| TEXAS INSTRUMENTS INCORPORATED
| Standard Linear and Logic Group
| IBIS Model of SN74AUC16244
| 16-Bit Bufer/Driver with 3-State Outputs
| This file contains package information for the following:
|  TSSOP 48-pin (DGG) package as [Component] AUC16244_DGG
|  TVSOP 48-pin (DGV) package as [component] AUC16244_DGV
|  VFBGA 56-PIN (GQL) PACKAGE AS [COMPONENT] AUC16244-GQL
| This device can be powered at the following Vccs:
|  2.5 volt Vcc
|  1.8 volt Vcc
|  1.5 volt Vcc
|  1.2 volt Vcc
|  0.8 volt Vcc
| This file provides unique models under the [Model Selector] for each Vcc.
| For operation at a specific Vcc, select the appropriate model after each
| [Model Selector] keyword.
[IBIS Ver]   3.2
[Comment char]  |_char
[File Name]   sn74auc16244.ibs
[File Rev]   1.1 | x_die
[Date]   May 23, 2002
[Source]   Data created from TI-SPICE simulations at TI-SLL.
[Notes]   The following is an IBIS list for the AUC16244.
   Please contact sllibis@ti.com with questions and
   comments concerning SLL IBIS models.
   -Power clamp data deleted as there is no power-clamp diode.
   -The waveforms for the AUC16244_OUT ,Pullup and
   Pulldown are caused by the circuitry that helps reduce
   overshoot and undershoot in transmission lines (EMI).
   These waveforms are norimal for this particular design.
   -End point warning due to AC and DC mismatch.
   -GQL package is package preview only at this date
[Disclaimer] Property of Texas Instruments Incorporated.  Unauthorized
   reproduction and/or distribution is strictly prohibited.
   This product is protected under copyright law.
   Created  2002, (C) Copyright  2002, Texas Instruments
   Incorporated, All Rights Reserved
   UNLESS THERE IS A SIGNED, WRITTEN AGREEMENT TO THE
   CONTRARY, TEXAS INSTRUMENTS (TI) IS PROVIDING THE IBIS
   MODELS  AND WITHOUT ANY WARRANTY, EXPRESSED OR
   IMPLIED.  TI assumes no liability for:
   1) the accuracy of the IBIS models provided to your
   company;
   2) the proper functioning of these IBIS Models in your
   design or for any resulting applications; or
   3) infringement of patents, copyrights or intellectual
   property rights resulting from your use of these IBIS
   models.
   TI provides IBIS Models as a service to our customers.
   You and your company shall not distribute, sell or give
   these models to anyone else without prior written
   permission from TI.
   TI reserves the right to make changes to our products or
   to discontinue any semiconductor product or service
   without notice, and advises our customers to obtain the
   latest version of relevant information to verify, before
   placing orders, that the information being relied on is
   current.
   Please be aware that your receipt and use of the IBIS
   information provided shall serve as acceptance of these
   terms and conditions.  If you do not accept these terms,
   you should return or destroy the IBIS models and any
   other accompanying information immediately.
| Component AUC16244_DGG 48-pin TSSOP
[Component]   AUC16244_DGG
[Manufacturer]   Texas Instruments, Inc.
[Package]
|   typ   min   max
R_pkg   6.200e-02   5.000e-02   7.800e-02
L_pkg   3.527e-09   3.128e-09   4.255e-09
C_pkg   5.300e-13   4.170e-13   6.850e-13
[Pin]   signal_name   model_name   R_pin   L_pin   C_pin
1   1NOE   AUC16244_OEIN   5.000e-02   4.250e-09   6.710e-13
2   1Y1   AUC16244_OUT   5.700e-02   3.956e-09   6.740e-13
3   1Y2   AUC16244_OUT   7.100e-02   3.922e-09   6.190e-13
4   GND   GND   7.800e-02   3.841e-09   6.180e-13
5   1Y3   AUC16244_OUT   5.600e-02   3.535e-09   5.550e-13
6   1Y4   AUC16244_OUT   5.800e-02   3.464e-09   5.030e-13
7   VCC   POWER   6.000e-02   3.362e-09   4.980e-13
8   2Y1   AUC16244_OUT   6.100e-02   3.293e-09   4.620e-13
9   2Y2   AUC16244_OUT   6.300e-02   3.240e-09   4.550e-13
10   GND   GND   6.300e-02   3.175e-09   4.420e-13
11   2Y3   AUC16244_OUT   6.400e-02   3.153e-09   4.290e-13
12   2Y4   AUC16244_OUT   6.500e-02   3.128e-09   4.180e-13
13   3Y1   AUC16244_OUT   6.500e-02   3.128e-09   4.180e-13
14   3Y2   AUC16244_OUT   6.400e-02   3.154e-09   4.290e-13
15   GND   GND   6.300e-02   3.174e-09   4.420e-13
16   3Y3   AUC16244_OUT   6.300e-02   3.241e-09   4.550e-13
17   3Y4   AUC16244_OUT   6.100e-02   3.293e-09   4.620e-13
18   VCC   POWER   6.000e-02   3.362e-09   4.970e-13
19   4Y1   AUC16244_OUT   5.800e-02   3.464e-09   5.030e-13
20   4Y2   AUC16244_OUT   5.600e-02   3.537e-09   5.600e-13
21   GND   GND   7.700e-02   3.839e-09   6.260e-13
22   4Y3   AUC16244_OUT   7.100e-02   3.917e-09   6.270e-13
23   4Y4   AUC16244_OUT   5.800e-02   3.955e-09   6.850e-13
24   4NOE   AUC16244_OEIN   5.200e-02   4.255e-09   6.790e-13
25   3NOE   AUC16244_OEIN   5.100e-02   4.254e-09   6.760e-13
26   4A4   AUC16244_AIN   5.800e-02   3.957e-09   6.790e-13
27   4A3   AUC16244_AIN   7.100e-02   3.920e-09   6.210e-13
28   GND   GND   7.800e-02   3.843e-09   6.220e-13
29   4A2   AUC16244_AIN   5.600e-02   3.539e-09   5.600e-13
30   4A1   AUC16244_AIN   5.800e-02   3.466e-09   5.030e-13
31   VCC   POWER   6.000e-02   3.363e-09   4.970e-13
32   3A4   AUC16244_AIN   6.100e-02   3.294e-09   4.620e-13
33   3A3   AUC16244_AIN   6.300e-02   3.241e-09   4.540e-13
34   GND   GND   6.300e-02   3.175e-09   4.410e-13
35   3A2   AUC16244_AIN   6.400e-02   3.153e-09   4.290e-13
36   3A1   AUC16244_AIN   6.500e-02   3.129e-09   4.170e-13
37   2A4   AUC16244_AIN   6.500e-02   3.129e-09   4.170e-13
38   2A3   AUC16244_AIN   6.400e-02   3.152e-09   4.290e-13
39   GND   GND   6.400e-02   3.176e-09   4.410e-13
40   2A2   AUC16244_AIN   6.300e-02   3.241e-09   4.540e-13
41   2A1   AUC16244_AIN   6.100e-02   3.293e-09   4.620e-13
42   VCC   POWER   6.000e-02   3.363e-09   4.970e-13
43   1A4   AUC16244_AIN   5.800e-02   3.464e-09   5.030e-13
44   1A3   AUC16244_AIN   5.600e-02   3.534e-09   5.610e-13
45   GND   GND   7.800e-02   3.841e-09   6.260e-13
46   1A2   AUC16244_AIN   7.100e-02   3.920e-09   6.220e-13
47   1A1   AUC16244_AIN   5.700e-02   3.955e-09   6.770e-13
48   2NOE   AUC16244_OEIN   5.100e-02   4.252e-09   6.720e-13
| Component AUC16244_DGV 48-pin TVSOP
[Component]   AUC16244_DGV
[Manufacturer] Texas Instruments, Inc.
[Package]
|   typ   min   max
R_pkg   7.000e-02   4.900e-02   8.500e-02
L_pkg   3.013e-09   2.743e-09   3.408e-09
C_pkg   3.710e-13   2.940e-13   5.110e-13
[Pin]   signal_name   model_name   R_pin   L_pin   C_pin
1   1NOE   AUC16244_OEIN   4.900e-02   3.393e-09   4.970e-13
2   1Y1   AUC16244_OUT   6.000e-02   3.250e-09   5.020e-13
3   1Y2   AUC16244_OUT   7.700e-02   3.310e-09   4.510e-13
4   GND   GND   8.500e-02   3.299e-09   4.040e-13
5   1Y3   AUC16244_OUT   8.300e-02   3.136e-09   3.600e-13
6   1Y4   AUC16244_OUT   7.700e-02   3.019e-09   3.630e-13
7   VCC   POWER   6.500e-02   2.882e-09   3.490e-13
8   2Y1   AUC16244_OUT   6.600e-02   2.829e-09   3.140e-13
9   2Y2   AUC16244_OUT   6.700e-02   2.796e-09   3.140e-13
10   GND   GND   6.900e-02   2.754e-09   3.080e-13
11   2Y3   AUC16244_OUT   7.000e-02   2.753e-09   3.010e-13
12   2Y4   AUC16244_OUT   7.100e-02   2.745e-09   2.940e-13
13   3Y1   AUC16244_OUT   7.000e-02   2.744e-09   2.940e-13
14   3Y2   AUC16244_OUT   7.000e-02   2.754e-09   3.010e-13
15   GND   GND   6.900e-02   2.754e-09   3.080e-13
16   3Y3   AUC16244_OUT   6.700e-02   2.796e-09   3.140e-13
17   3Y4   AUC16244_OUT   6.600e-02   2.829e-09   3.140e-13
18   VCC   POWER   6.500e-02   2.883e-09   3.500e-13
19   4Y1   AUC16244_OUT   7.500e-02   3.014e-09   3.630e-13
20   4Y2   AUC16244_OUT   8.000e-02   3.128e-09   3.580e-13
21   GND   GND   8.400e-02   3.295e-09   4.030e-13
22   4Y3   AUC16244_OUT   7.800e-02   3.311e-09   4.520e-13
23   4Y4   AUC16244_OUT   6.200e-02   3.259e-09   5.010e-13
24   4NOE   AUC16244_OEIN   5.200e-02   3.404e-09   4.960e-13
25   3NOE   AUC16244_OEIN   5.300e-02   3.397e-09   5.050e-13
26   4A4   AUC16244_AIN   6.200e-02   3.249e-09   5.110e-13
27   4A3   AUC16244_AIN   7.700e-02   3.308e-09   4.530e-13
28   GND   GND   8.200e-02   3.289e-09   4.030e-13
29   4A2   AUC16244_AIN   7.800e-02   3.121e-09   3.590e-13
30   4A1   AUC16244_AIN   7.400e-02   3.010e-09   3.630e-13
31   VCC   POWER   6.500e-02   2.883e-09   3.490e-13
32   3A4   AUC16244_AIN   6.700e-02   2.829e-09   3.140e-13
33   3A3   AUC16244_AIN   6.700e-02   2.795e-09   3.140e-13
34   GND   GND   6.900e-02   2.753e-09   3.070e-13
35   3A2   AUC16244_AIN   7.000e-02   2.753e-09   3.010e-13
36   3A1   AUC16244_AIN   7.000e-02   2.743e-09   2.940e-13
37   2A4   AUC16244_AIN   7.000e-02   2.743e-09   2.940e-13
38   2A3   AUC16244_AIN   7.000e-02   2.753e-09   3.010e-13
39   GND   GND   6.900e-02   2.754e-09   3.070e-13
40   2A2   AUC16244_AIN   6.800e-02   2.797e-09   3.140e-13
41   2A1   AUC16244_AIN   6.700e-02   2.830e-09   3.140e-13
42   VCC   POWER   6.400e-02   2.880e-09   3.490e-13
43   1A4   AUC16244_AIN   7.200e-02   3.004e-09   3.620e-13
44   1A3   AUC16244_AIN   7.800e-02   3.121e-09   3.590e-13
45   GND   GND   8.400e-02   3.296e-09   4.030e-13
46   1A2   AUC16244_AIN   7.700e-02   3.308e-09   4.510e-13
47   1A1   AUC16244_AIN   6.200e-02   3.258e-09   4.990e-13
48   2NOE   AUC16244_OEIN   5.300e-02   3.408e-09   4.940e-13
|   VFBGA PACKAGE (GQL)
[Component]   AUC16244_GQL
[manufacturer]   Texas Instruments, Inc.
[Package]
|   typ   min   max
R_pkg   0.065   0.035   0.097
L_pkg   1.952nH   1.000nH   3.191nH
C_pkg   0.283pF   0.162pF   0.434pF
[Pin] signal_name   model_name   R_pin   L_pin   C_pin
A3   NC   NC   0.036   1.004nH   0.176pF
A2   NC   NC   0.04   1.191nH   0.186pF
A1   1OEIN   AUC16244_OEIN   0.047   1.411nH   0.209pF
B3   GND   GND   0.097   3.191nH   0.434pF
B2   1Y1   AUC16244_OUT   0.074   2.213nH   0.329pF
B1   1Y2   AUC16244_AIN   0.06   1.712nH   0.243pF
C3   VCC   POWER   0.085   2.691nH   0.368pF
C2   1Y3   AUC16244_AIN   0.074   2.16nH   0.315pF
C1   1Y4   AUC16244_AIN   0.06   1.666nH   0.247pF
D2   2Y1   AUC16244_AIN   0.074   2.121nH   0.313pF
D3   GND   GND   0.091   2.924nH   0.397pF
D1   2Y2   AUC16244_AIN   0.06   1.619nH   0.245pF
E2   2Y3   AUC16244_AIN   0.069   2.031nH   0.288pF
E1   2Y4   AUC16244_AIN   0.06   1.583nH   0.22pF
F1   3Y1   AUC16244_AIN   0.06   1.578nH   0.22pF
F2   3Y2   AUC16244_AIN   0.069   2.017nH   0.286pF
G1   3Y3   AUC16244_AIN   0.06   1.594nH   0.241pF
G3   GND   GND   0.092   2.917nH   0.397pF
G2   3Y4   AUC16244_OUT   0.075   2.114nH   0.315pF
H1   4Y1   AUC16244_OUT   0.06   1.632nH   0.247pF
H2   4Y2   AUC16244_OUT   0.07   2.074nH   0.307pF
H3   VCC   POWER   0.086   2.664nH   0.365pF
J1   4Y3   AUC16244_OUT   0.06   1.689nH   0.249pF
J2   4Y4   AUC16244_OUT   0.066   2.152nH   0.332pF
J3   GND   GND   0.087   3.118nH   0.423pF
K1   4OEIN   AUC16244_OEIN   0.038   1.303nH   0.2pF
K2   NC   NC   0.035   1.176nH   0.183pF
K3   NC   NC   0.035   1.007nH   0.162pF
K4   NC   NC   0.035   1nH   0.162pF
K5   NC   NC   0.035   1.154nH   0.18pF
K6   3OEIN   AUC16244_OEIN   0.041   1.352nH   0.204pF
J4   GND   GND   0.088   3.137nH   0.43pF
J5   4A4   AUC16244_AIN   0.074   2.218nH   0.334pF
J6   4A3   AUC16244_AIN   0.06   1.683nH   0.25pF
H4   VCC   POWER   0.085   2.658nH   0.372pF
H5   4A2   AUC16244_AIN   0.075   2.149nH   0.321pF
H6   4A1   AUC16244_AIN   0.06   1.627nH   0.248pF
G5   3A4   AUC16244_AIN   0.075   2.113nH   0.314pF
G4   GND   GND   0.092   2.922nH   0.396pF
G6   3A3   AUC16244_AIN   0.06   1.594nH   0.242pF
F5   3A2   AUC16244_AIN   0.069   2.016nH   0.288pF
F6   3A1   AUC16244_AIN   0.06   1.58nH   0.221pF
E6   2A4   AUC16244_AIN   0.06   1.582nH   0.22pF
E5   2A3   AUC16244_AIN   0.069   2.026nH   0.289pF
D6   2A2   AUC16244_AIN   0.06   1.61nH   0.245pF
D4   GND   GND   0.092   2.933nH   0.396pF
D5   2A1   AUC16244_AIN   0.075   2.126nH   0.311pF
C6   1A4   AUC16244_AIN   0.06   1.641nH   0.245pF
C5   1A3   AUC16244_AIN   0.073   2.168nH   0.319pF
C4   VCC   POWER   0.086   2.675nH   0.362pF
B6   1A2   AUC16244_AIN   0.06   1.688nH   0.243pF
B5   1A1   AUC16244_AIN   0.075   2.281nH   0.333pF
B4   GND   GND   0.095   3.168nH   0.424pF
A6   2OEIN   AUC16244_AIN   0.045   1.418nH   0.209pF
A5   NC   NC   0.039   1.216nH   0.19pF
A4   NC   NC   0.037   1.029nH   0.179pF
| Model AUC16244_AIN
[Model Selector]   AUC16244_AIN
AUC16244_AIN_25   2.5 volt Vcc
AUC16244_AIN_18   1.8 volt Vcc
AUC16244_AIN_15A   1.5 volt Vcc
AUC16244_AIN_12   1.2 volt Vcc
AUC16244_AIN_08   0.8 volt Vcc
| Model AUC16244_OEIN
[Model Selector]   AUC16244_OEIN
AUC16244_OEIN_25   2.5 volt Vcc
AUC16244_OEIN_18   1.8 volt Vcc
AUC16244_OEIN_15A   1.5 volt Vcc
AUC16244_OEIN_12   1.2 volt Vcc
AUC16244_OEIN_08   0.8 volt Vcc
| Model AUC16244_OUT
[Model Selector]   AUC16244_OUT
AUC16244_OUT_25   2.5 volt Vcc
AUC16244_OUT_18   1.8 volt Vcc
AUC16244_OUT_15A   1.5 volt Vcc
AUC16244_OUT_12   1.2 volt Vcc
AUC16244_OUT_08   0.8 volt Vcc
| Models and submodels in the file (15): AUC16244_AIN_25 (Input), AUC16244_AIN_18 (Input), AUC16244_AIN_15A (Input), AUC16244_AIN_12 (Input), AUC16244_AIN_08 (Input), AUC16244_OEIN_25 (Input), AUC16244_OEIN_18 (Input), AUC16244_OEIN_15A (Input), AUC16244_OEIN_12 (Input), AUC16244_OEIN_08 (Input), AUC16244_OUT_25 (3-state), AUC16244_OUT_18 (3-state), AUC16244_OUT_15A (3-state), AUC16244_OUT_12 (3-state), AUC16244_OUT_08 (3-state)
